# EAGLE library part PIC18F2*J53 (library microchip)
PIC18F47J53 Family High-Performance USB Microcontrollers with nanoWatt XLP Technology Source: Data sheet
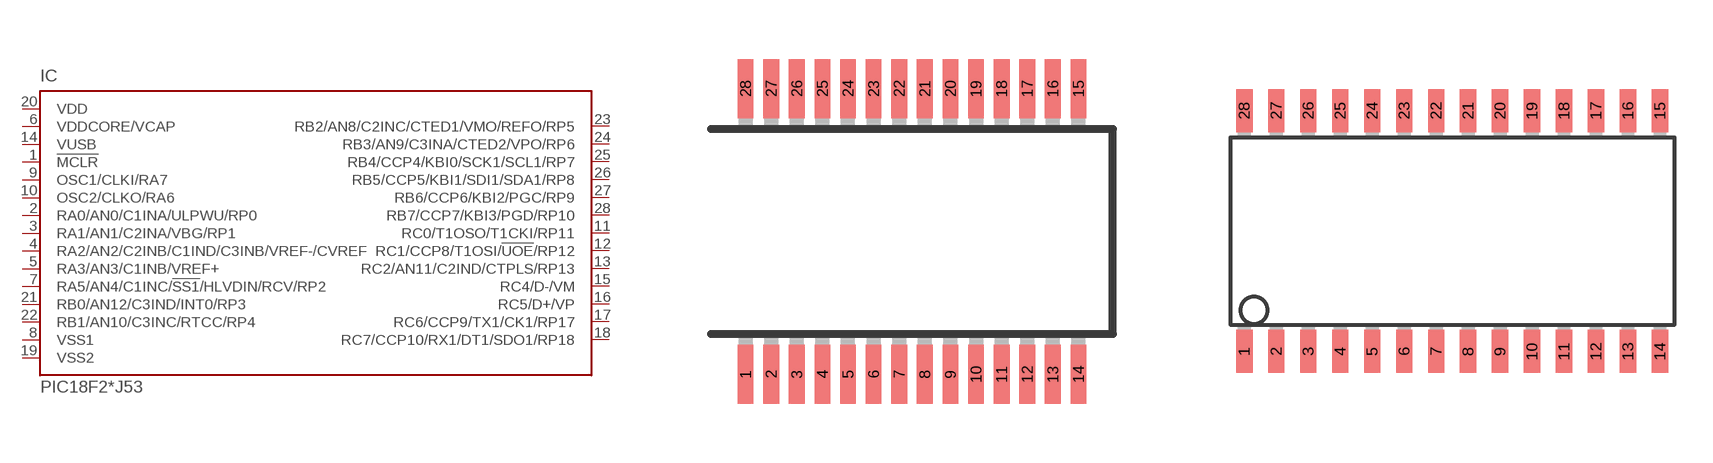
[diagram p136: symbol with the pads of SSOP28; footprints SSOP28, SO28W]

Designator prefix IC

## PIC18F26J53SS (OC_FARNELL: unknown; OC_NEWARK: unknown), PIC18F27J53SS (OC_FARNELL: unknown; OC_NEWARK: unknown)  [SSOP28]
1  !MCLR  in
2  RA0/AN0/C1INA/ULPWU/RP0
3  RA1/AN1/C2INA/VBG/RP1
4  RA2/AN2/C2INB/C1IND/C3INB/VREF-/CVREF
5  RA3/AN3/C1INB/VREF+
6  VDDCORE/VCAP  in
7  RA5/AN4/C1INC/!SS1!/HLVDIN/RCV/RP2
8  VSS1  in
9  OSC1/CLKI/RA7
10  OSC2/CLKO/RA6
11  RC0/T1OSO/T1CKI/RP11
12  RC1/CCP8/T1OSI/!UOE!/RP12
13  RC2/AN11/C2IND/CTPLS/RP13
14  VUSB  in
15  RC4/D-/VM
16  RC5/D+/VP
17  RC6/CCP9/TX1/CK1/RP17
18  RC7/CCP10/RX1/DT1/SDO1/RP18
19  VSS2  in
20  VDD  in
21  RB0/AN12/C3IND/INT0/RP3
22  RB1/AN10/C3INC/RTCC/RP4
23  RB2/AN8/C2INC/CTED1/VMO/REFO/RP5
24  RB3/AN9/C3INA/CTED2/VPO/RP6
25  RB4/CCP4/KBI0/SCK1/SCL1/RP7
26  RB5/CCP5/KBI1/SDI1/SDA1/RP8
27  RB6/CCP6/KBI2/PGC/RP9
28  RB7/CCP7/KBI3/PGD/RP10

## PIC18F26J53SO (MPN: PIC18F26J53-I/SO; OC_FARNELL: unknown; OC_NEWARK: 63R7830), PIC18F27J53SO (MPN: PIC18F27J53-I/SO; OC_FARNELL: unknown; OC_NEWARK: 63R7838)  [SO28W]
Pads as for SSOP28

## PIC18F26J53ML (MPN: PIC18F26J53-I/ML; OC_FARNELL: unknown; OC_NEWARK: 63R7829), PIC18F27J53ML (MPN: PIC18F27J53-I/ML; OC_FARNELL: 1814994; OC_NEWARK: 63R7837)  [QFN28-ML_6X6MM]
1  RA2/AN2/C2INB/C1IND/C3INB/VREF-/CVREF
2  RA3/AN3/C1INB/VREF+
3  VDDCORE/VCAP  in
4  RA5/AN4/C1INC/!SS1!/HLVDIN/RCV/RP2
5  VSS1  in
6  OSC1/CLKI/RA7
7  OSC2/CLKO/RA6
8  RC0/T1OSO/T1CKI/RP11
9  RC1/CCP8/T1OSI/!UOE!/RP12
10  RC2/AN11/C2IND/CTPLS/RP13
11  VUSB  in
12  RC4/D-/VM
13  RC5/D+/VP
14  RC6/CCP9/TX1/CK1/RP17
15  RC7/CCP10/RX1/DT1/SDO1/RP18
16  VSS2  in
17  VDD  in
18  RB0/AN12/C3IND/INT0/RP3
19  RB1/AN10/C3INC/RTCC/RP4
20  RB2/AN8/C2INC/CTED1/VMO/REFO/RP5
21  RB3/AN9/C3INA/CTED2/VPO/RP6
22  RB4/CCP4/KBI0/SCK1/SCL1/RP7
23  RB5/CCP5/KBI1/SDI1/SDA1/RP8
24  RB6/CCP6/KBI2/PGC/RP9
25  RB7/CCP7/KBI3/PGD/RP10
26  !MCLR  in
27  RA0/AN0/C1INA/ULPWU/RP0
28  RA1/AN1/C2INA/VBG/RP1

## PIC18F26J53SP (MPN: PIC18F26J53-I/SP; OC_FARNELL: unknown; OC_NEWARK: 63R7831), PIC18F27J53SP (MPN: PIC18F27J53-I/SP; OC_FARNELL: unknown; OC_NEWARK: 63R7839)  [DIL28-3]
Pads as for SSOP28

## Footprint SSOP28 (pad centres in mm)
Shrink Small Outline Package package type SS
smd 0.4 x 1.5: 1 -4.225,-3.625; 2 -3.575,-3.625; 3 -2.925,-3.625; 4 -2.275,-3.625; 5 -1.625,-3.625; 6 -0.975,-3.625; 7 -0.325,-3.625; 8 0.325,-3.625; 9 0.975,-3.625; 10 1.625,-3.625; 11 2.275,-3.625; 12 2.925,-3.625; 13 3.575,-3.625; 14 4.225,-3.625; 15 4.225,3.625; 16 3.575,3.625; 17 2.925,3.625; 18 2.275,3.625; 19 1.625,3.625; 20 0.975,3.625; 21 0.325,3.625; 22 -0.325,3.625; 23 -0.975,3.625; 24 -1.625,3.625; 25 -2.275,3.625; 26 -2.925,3.625; 27 -3.575,3.625; 28 -4.225,3.625

## Footprint SO28W (pad centres in mm)
28-Lead Plastic Small Outline (SO) Wide, 300 mil Body (SOIC) Source: http://ww1.microchip.com/downloads/en/devicedoc/39632c.pdf
smd 0.65 x 1.7: 1 -7.62,-4.78; 2 -6.35,-4.78; 3 -5.08,-4.78; 4 -3.81,-4.78; 5 -2.54,-4.78; 6 -1.27,-4.78; 7 0,-4.78; 8 1.27,-4.78; 9 2.54,-4.78; 10 3.81,-4.78; 11 5.08,-4.78; 12 6.35,-4.78; 13 7.62,-4.78; 14 8.89,-4.78; 15 8.89,4.78; 16 7.62,4.78; 17 6.35,4.78; 18 5.08,4.78; 19 3.81,4.78; 20 2.54,4.78; 21 1.27,4.78; 22 0,4.78; 23 -1.27,4.78; 24 -2.54,4.78; 25 -3.81,4.78; 26 -5.08,4.78; 27 -6.35,4.78; 28 -7.62,4.78

## Footprint QFN28-ML_6X6MM (pad centres in mm)
QFN28-ML_6X6MM Source: http://www.microchip.com .. 39637a.pdf
smd 0.7 x 0.35: 1 -2.7,1.95; 2 -2.7,1.3; 3 -2.7,0.65; 4 -2.7,0; 5 -2.7,-0.65; 6 -2.7,-1.3; 7 -2.7,-1.95; 15 2.7,-1.95; 16 2.7,-1.3; 17 2.7,-0.65; 18 2.7,0; 19 2.7,0.65; 20 2.7,1.3; 21 2.7,1.95
smd 0.35 x 0.7: 8 -1.95,-2.7; 9 -1.3,-2.7; 10 -0.65,-2.7; 11 0,-2.7; 12 0.65,-2.7; 13 1.3,-2.7; 14 1.95,-2.7; 22 1.95,2.7; 23 1.3,2.7; 24 0.65,2.7; 25 0,2.7; 26 -0.65,2.7; 27 -1.3,2.7; 28 -1.95,2.7
smd 3.7 x 3.7: EXP 0,0

## Footprint DIL28-3 (pad centres in mm)
Dual In Line package type P
drill 0.813 long: 1 -16.51,-3.81; 2 -13.97,-3.81; 3 -11.43,-3.81; 4 -8.89,-3.81; 5 -6.35,-3.81; 6 -3.81,-3.81; 7 -1.27,-3.81; 8 1.27,-3.81; 9 3.81,-3.81; 10 6.35,-3.81; 11 8.89,-3.81; 12 11.43,-3.81; 13 13.97,-3.81; 14 16.51,-3.81; 15 16.51,3.81; 16 13.97,3.81; 17 11.43,3.81; 18 8.89,3.81; 19 6.35,3.81; 20 3.81,3.81; 21 1.27,3.81; 22 -1.27,3.81; 23 -3.81,3.81; 24 -6.35,3.81; 25 -8.89,3.81; 26 -11.43,3.81; 27 -13.97,3.81; 28 -16.51,3.81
